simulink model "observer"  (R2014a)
settings: Solver=ode45  StartTime=0.0  StopTime=tend  RelTol=1e-3
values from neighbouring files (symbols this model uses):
  A = [0 1; 0 0]    [L9.m]    (also in L9_LandObs_script.m; L9_fullExample_script.m; L9_onlyL_script.m)
  B = [0; 1]    [L9.m]    (also in L9_LandObs_script.m; L9_fullExample_script.m; L9_onlyL_script.m)
  C = [1, 0]    [L9.m]    (also in L9_LandObs_script.m; L9_fullExample_script.m; L9_onlyL_script.m)
  Cx = eye(size(A))    [L9.m]    (also in L9_LandObs_script.m; L9_fullExample_script.m; L9_onlyL_script.m)
  Dx = zeros(size(Cx,1),size(B,2))    [L9.m]    (also in L9_LandObs_script.m; L9_fullExample_script.m; L9_onlyL_script.m)
  Gamma = Gamma3    [L9.m]
  h = h3    (= 0.5)    [L9.m]    (also in L9_LandObs_script.m = 0.44; L9_fullExample_script.m = 0.44; L9_onlyL_script.m = 0.44)
  K = Kdb3    [L9.m]    (also in L9_LandObs_script.m = acker(Phi',C',p_obs)'; L9_fullExample_script.m = Ke(1:size(Phi,1)))
  L = L3    [L9.m]    (also in L9_LandObs_script.m = place(Phi,Gamma,pd); L9_fullExample_script.m = place(Phi,Gamma,pd); L9_onlyL_script.m = place(Phi,Gamma,pd))
  Phi = Phi3    [L9.m]
  x0 = [1;1]    [L9.m]    (also in L9_LandObs_script.m; L9_fullExample_script.m; L9_onlyL_script.m)

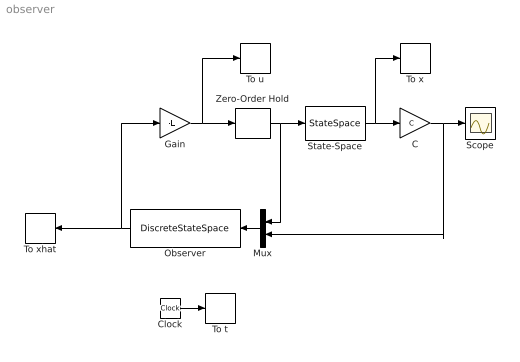
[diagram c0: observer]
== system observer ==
  C : Gain  Gain=C  Multiplication=Matrix(K*u)  SampleTime=h
  Clock : Clock
  Gain : Gain  Gain=-L  Multiplication=Matrix(K*u)  SampleTime=h
  Mux : Mux  Inputs=2
  Observer : DiscreteStateSpace  A=Phi-K*C  B=[Gamma,K]  C=eye(size(Phi))  D=zeros(2,2)  SampleTime=h
  Scope : Scope
  State-Space : StateSpace  A=A  B=B  C=Cx  D=Dx  X0=x0
  To t : ToWorkspace  VariableName=t  SampleTime=h
  To u : ToWorkspace  VariableName=u  SampleTime=h
  To x : ToWorkspace  VariableName=x  SampleTime=h
  To xhat : ToWorkspace  VariableName=xhat  SampleTime=h
  Zero-Order Hold : ZeroOrderHold  SampleTime=h
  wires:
  Zero-Order Hold/1 -> Mux/1, State-Space/1
  Gain/1 -> To u/1, Zero-Order Hold/1
  State-Space/1 -> C/1, To x/1
  Clock/1 -> To t/1
  Mux/1 -> Observer/1
  Observer/1 -> To xhat/1, Gain/1
  C/1 -> Mux/2, Scope/1
